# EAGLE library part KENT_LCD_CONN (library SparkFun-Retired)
Connector for Kent display (LCD-09560) SparkFun no longer uses this connector on any active designs, however 4Ucon still makes this connector as of 7/19/2016. http://www.4uconnector.com/online/object/4udrawing/07612.pdf
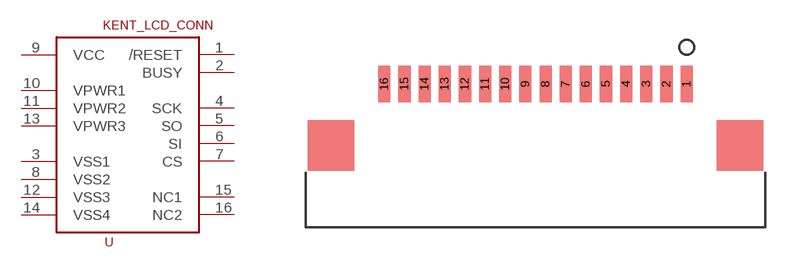
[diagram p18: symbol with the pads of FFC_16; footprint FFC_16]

Designator prefix -

## KENT_LCD_CONN  [FFC_16]
1  /RESET
2  BUSY
3  VSS1
4  SCK
5  SO
6  SI
7  CS
8  VSS2
9  VCC
10  VPWR1
11  VPWR2
12  VSS3
13  VPWR3
14  VSS4
15  NC1
16  NC2

## Footprint FFC_16 (pad centres in mm)
smd 0.6 x 1.8: 1 7.5,3.9; 2 6.5,3.9; 3 5.5,3.9; 4 4.5,3.9; 5 3.5,3.9; 6 2.5,3.9; 7 1.5,3.9; 8 0.5,3.9; 9 -0.5,3.9; 10 -1.5,3.9; 11 -2.5,3.9; 12 -3.5,3.9; 13 -4.5,3.9; 14 -5.5,3.9; 15 -6.5,3.9; 16 -7.5,3.9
